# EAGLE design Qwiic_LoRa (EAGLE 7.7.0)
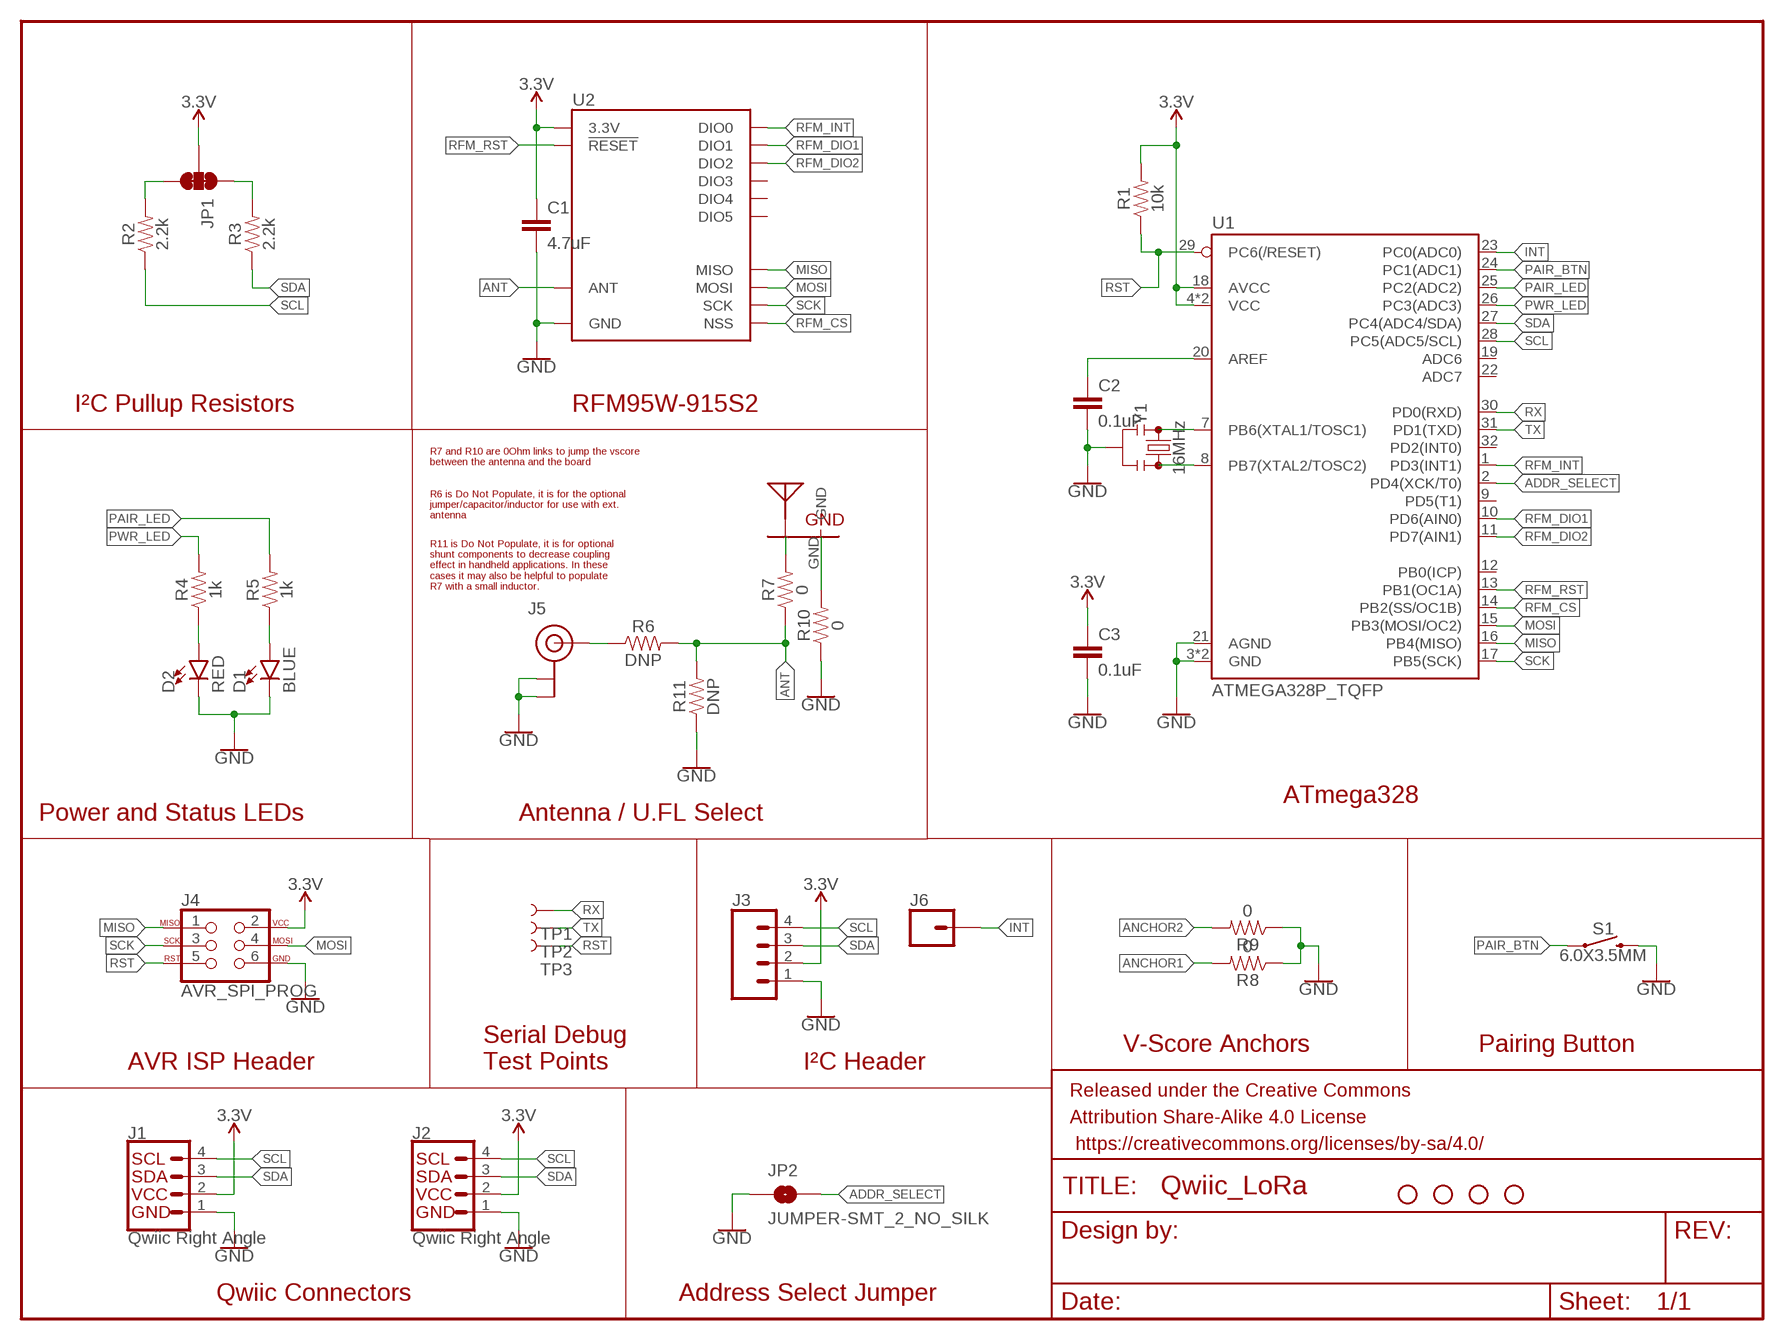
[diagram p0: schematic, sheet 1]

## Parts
C1  4.7uF  4.7UF0603  [0603]
C2  0.1uF  0.1UF-0603-25V-(+80/-20%)  [0603]
C3  0.1uF  0.1UF-0603-25V-(+80/-20%)  [0603]
D1  BLUE  LED-BLUE0603  [LED-0603]
D2  RED  LED-RED0603  [LED-0603]
FRAME1  FRAME-LETTER  [CREATIVE_COMMONS]
H1  STAND-OFF  [STAND-OFF]
H2  STAND-OFF  [STAND-OFF]
H3  STAND-OFF  [STAND-OFF]
H4  STAND-OFF  [STAND-OFF]
J1  Qwiic Right Angle  I2C_STANDARDQWIIC  [1X04_1MM_RA]
J2  Qwiic Right Angle  I2C_STANDARDQWIIC  [1X04_1MM_RA]
J3  CONN_041X04_NO_SILK  [1X04_NO_SILK]
J4  AVR_SPI_PROG  AVR_SPI_PROG_3X2TESTPOINTS  [2X3_TEST_POINTS]
J5  U.FL  [U.FL]
J6  CONN_01PTH_NO_SILK_YES_STOP  [1X01_NO_SILK]
JP1  JUMPER-SMT_3_2-NC_TRACE_SILK  [SMT-JUMPER_3_2-NC_TRACE_SILK]
JP2  JUMPER-SMT_2_NO_SILK  [SMT-JUMPER_2_NO_SILK]
R1  10k  10KOHM-0603-1/10W-1%  [0603]
R2  2.2k  2.2KOHM-0603-1/10W-1%  [0603]
R3  2.2k  2.2KOHM-0603-1/10W-1%  [0603]
R4  1k  1KOHM-0603-1/10W-1%  [0603]
R5  1k  1KOHM-0603-1/10W-1%  [0603]
R6  DNP  RESISTOR0603  [0603]
R7  0  RESISTOR0603  [0603]
R8  0  RESISTOR0603  [0603]
R9  0  RESISTOR0603  [0603]
R10  0  RESISTOR0603  [0603]
R11  DNP  RESISTOR0603  [0603]
S1  6.0X3.5MM  MOMENTARY-SWITCH-SPST-SMD-6.0X3.5MM  [TACTILE_SWITCH_SMD_6.0X3.5MM]
TP1  TEST-POINT3  [PAD.03X.03]
TP2  TEST-POINT3  [PAD.03X.03]
TP3  TEST-POINT3  [PAD.03X.03]
U1  ATMEGA328P_TQFP  [TQFP32-08]
U2  RFM96W  [RFM95/96/97/98W]
U$1  ANTENNA_915MHZ_INVERTED_F  [ANTENNA_INVERTED_F_915MHZ]
Y1  16MHz  RESONATOR-16MHZSMD_3.2X1.3  [RESONATOR-SMD-3.2X1.3]

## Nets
3.3V [3v3]: C1.1 C3.1 J1.2 J2.2 J3.2 J4.2 JP1.2 R1.2 U1.4(VCC) U1.6(VCC) U1.18(AVCC) U2.3.3V
ADDR_SELECT: JP2.2 U1.2(PD4(XCK/T0))
ANCHOR1: R8.2
ANCHOR2: R9.2
ANT: R6.2 R7.1 R11.2 U2.ANT
GND: C1.2 C2.2 C3.2 D1.C D2.C J1.1 J2.1 J3.1 J4.6 J5.1(GND) J5.2(GND) JP2.1 R8.1 R9.1 R10.1 R11.1 S1.2 U1.3(GND) U1.5(GND) U1.21(AGND) U2.GND@1(GND) U2.GND@2(GND) U2.GND@3(GND) Y1.2
INT: J6.1 U1.23(PC0(ADC0))
MISO: J4.1 U1.16(PB4(MISO)) U2.MISO
MOSI: J4.4 U1.15(PB3(MOSI/OC2)) U2.MOSI
N$1: D2.A R4.1
N$2: D1.A R5.1
N$3: C2.1 U1.20(AREF)
N$4: U1.7(PB6(XTAL1/TOSC1)) Y1.1
N$5: U1.8(PB7(XTAL2/TOSC2)) Y1.3
N$6: R7.2 U$1.FEED
N$7: JP1.1 R3.2
N$8: JP1.3 R2.2
N$9: J5.FEED(SIGNAL) R6.1
N$11: R10.2 U$1.GND
PAIR_BTN: S1.1 U1.24(PC1(ADC1))
PAIR_LED: R5.2 U1.25(PC2(ADC2))
PWR_LED: R4.2 U1.26(PC3(ADC3))
RFM_CS: U1.14(PB2(SS/OC1B)) U2.NSS
RFM_DIO1: U1.10(PD6(AIN0)) U2.DIO1
RFM_DIO2: U1.11(PD7(AIN1)) U2.DIO2
RFM_INT: U1.1(PD3(INT1)) U2.DIO0
RFM_RST: U1.13(PB1(OC1A)) U2.!RESET
RST: J4.5 R1.1 TP3.P$1 U1.29(PC6(/RESET))
RX: TP1.P$1 U1.30(PD0(RXD))
SCK: J4.3 U1.17(PB5(SCK)) U2.SCK
SCL: J1.4 J2.4 J3.4 R2.1 U1.28(PC5(ADC5/SCL))
SDA: J1.3 J2.3 J3.3 R3.1 U1.27(PC4(ADC4/SDA))
TX: TP2.P$1 U1.31(PD1(TXD))
Unconnected: U1.9(PD5(T1)) U1.12(PB0(ICP)) U1.19(ADC6) U1.22(ADC7) U1.32(PD2(INT0)) U2.DIO3 U2.DIO4 U2.DIO5

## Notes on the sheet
- I²C Pullup Resistors | RFM95W-915S2
- R7 and R10 are 0Ohm links to jump the vscore 
  between the antenna and the board
- R6 is Do Not Populate, it is for the optional 
  jumper/capacitor/inductor for use with ext.
  antenna
- R11 is Do Not Populate, it is for optional 
  shunt components to decrease coupling 
  effect in handheld applications. In these 
  cases it may also be helpful to populate 
  R7 with a small inductor.
- ATmega328
- Power and Status LEDs | Antenna / U.FL Select
- V-Score Anchors | Pairing Button
- AVR ISP Header
- Serial Debug
  Test Points
- I²C Header
- Qwiic Connectors | Address Select Jumper

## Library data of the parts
C1 = SparkFun-Capacitors:4.7UF: 4.7µF ceramic capacitors; PROD_ID: CAP-08280
C2 C3 = SparkFun-Capacitors:0.1UF: 0.1µF ceramic capacitors; PROD_ID: CAP-00810
D1 = SparkFun-LED:LED-BLUE: Blue SMD LED; PROD_ID: DIO-08575
D2 = SparkFun-LED:LED-RED: Red SMD LED; PROD_ID: DIO-00819
FRAME1 = SparkFun-Aesthetics:FRAME-LETTER: Schematic Frame - Letter
H1-H4 = SparkFun-Hardware:STAND-OFF: Stand Off
J1 J2 = SparkFun-Connectors:I2C_STANDARD: SparkFun I2C Standard Pinout Header SparkFun has standardized on a pinout for all I2C based sensor breakouts. This pinout allows I2C boards to be plugged directly into the headers on Arduino Uno compatible boards, and to be daisy chained easily. Example SparkFun Products: SparkFun Atmospheric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; PROD_ID: CONN-13694
J3 = SparkFun-Connectors:CONN_04: Multi connection point. Often used as Generic Header-pin footprint for 0.1 inch spaced/style header connections On any of the 0.1 inch spaced packages, you can populate with these: Break Away Headers - Straight (PRT-00116) Break Away Male Headers - Right Angle (PRT-00553) Female Headers (PRT-00115)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; PROD_ID: CONN-09696
J4 = SparkFun-Connectors:AVR_SPI_PROG_3X2: AVR ISP 6 Pin This is the reduced ISP connector for AVR programming. Common on Arduino. This footprint will take up less PCB space and can be used with a 10-pin to 6-pin adapter such as SKU: BOB-08508 **Special note about "TEST_POINT" package. The stop mask is on the top side, so if you want your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
J5 = SparkFun-Connectors:U.FL: SMD Antenna Connector - U.FL 2mm height, 3.0mm x 3.0mm receptacle size. SparkFun Products: SparkFun WiFi Shield - ESP8266 SparkFun ESP8266 Thing SparkFun MiniGen - Pro Mini Signal Generator Shield; PROD_ID: CONN-09193; SF_ID: WRL-09144
J6 = SparkFun-Connectors:CONN_01: Single connection point. Often used as Generic Header-pin footprint for 0.1 inch spaced/style header connections
JP1 = SparkFun-Jumpers:JUMPER-SMT_3_2-NC_TRACE: Normally closed trace jumper (2 of 2 connections) This jumper has a trace between all three pads so they are normally closed (NC). Use a razor knife to open the connection(s). For best results follow the IPC guidelines for cutting traces: Cutout at least 0.063 mm (0.005 in). Remove all loose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
JP2 = SparkFun-Jumpers:JUMPER-SMT_2_NO: Normally open jumper
R1 = SparkFun-Resistors:10KOHM: 10kΩ resistor; PROD_ID: RES-00824
R2 R3 = SparkFun-Resistors:2.2KOHM: 2.2kΩ resistor; PROD_ID: RES-08272
R4 R5 = SparkFun-Resistors:1KOHM: 1kΩ resistor; PROD_ID: RES-07856
R6-R11 = SparkFun-Resistors:RESISTOR: Generic Resistor Package
S1 = SparkFun-Switches:MOMENTARY-SWITCH-SPST: Momentary Switch (Pushbutton) - SPST; PROD_ID: SWCH-00815; SF_SKU: COM-08229
TP1-TP3 = SparkFun-Connectors:TEST-POINT: SparkFun Test Points
U1 = SparkFun-IC-Microcontroller:ATMEGA328P_TQFP: Popular 328P in QFP Storefront component: ATmega328 - TQFP (COM-13448) Datasheet SparkFun Products SparkFun RedBoard - Programmed with Arduino (DEV-12757) Arduino Pro Mini 328 - 5V/16MHz (DEV-11113) Arduino Pro Mini 328 - 3.3V/8MHz (DEV-11114) SparkFun OpenLog (DEV-13712) SparkFun MicroView - OLED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; PROD_ID: IC-09069
U2 = SparkX:RFM96W
U$1 = SparkX:ANTENNA_915MHZ_INVERTED_F
Y1 = SparkFun-Clocks:RESONATOR-16MHZ: 16MHz Resonator Digikey Example Frequency: 16MHz Frequency Stability: &plusmn;0.3% Frequency Tolerance: &plusmn;0.5% Capacitance: 15pF SparkFun Products SparkFun OpenLog SparkFun MicroView - OLED Arduino Module; PROD_ID: XTAL-08900

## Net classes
0 default: width 0.152 mm, drill 0.305 mm
1 3v3: width 0.203 mm, drill 0.305 mm

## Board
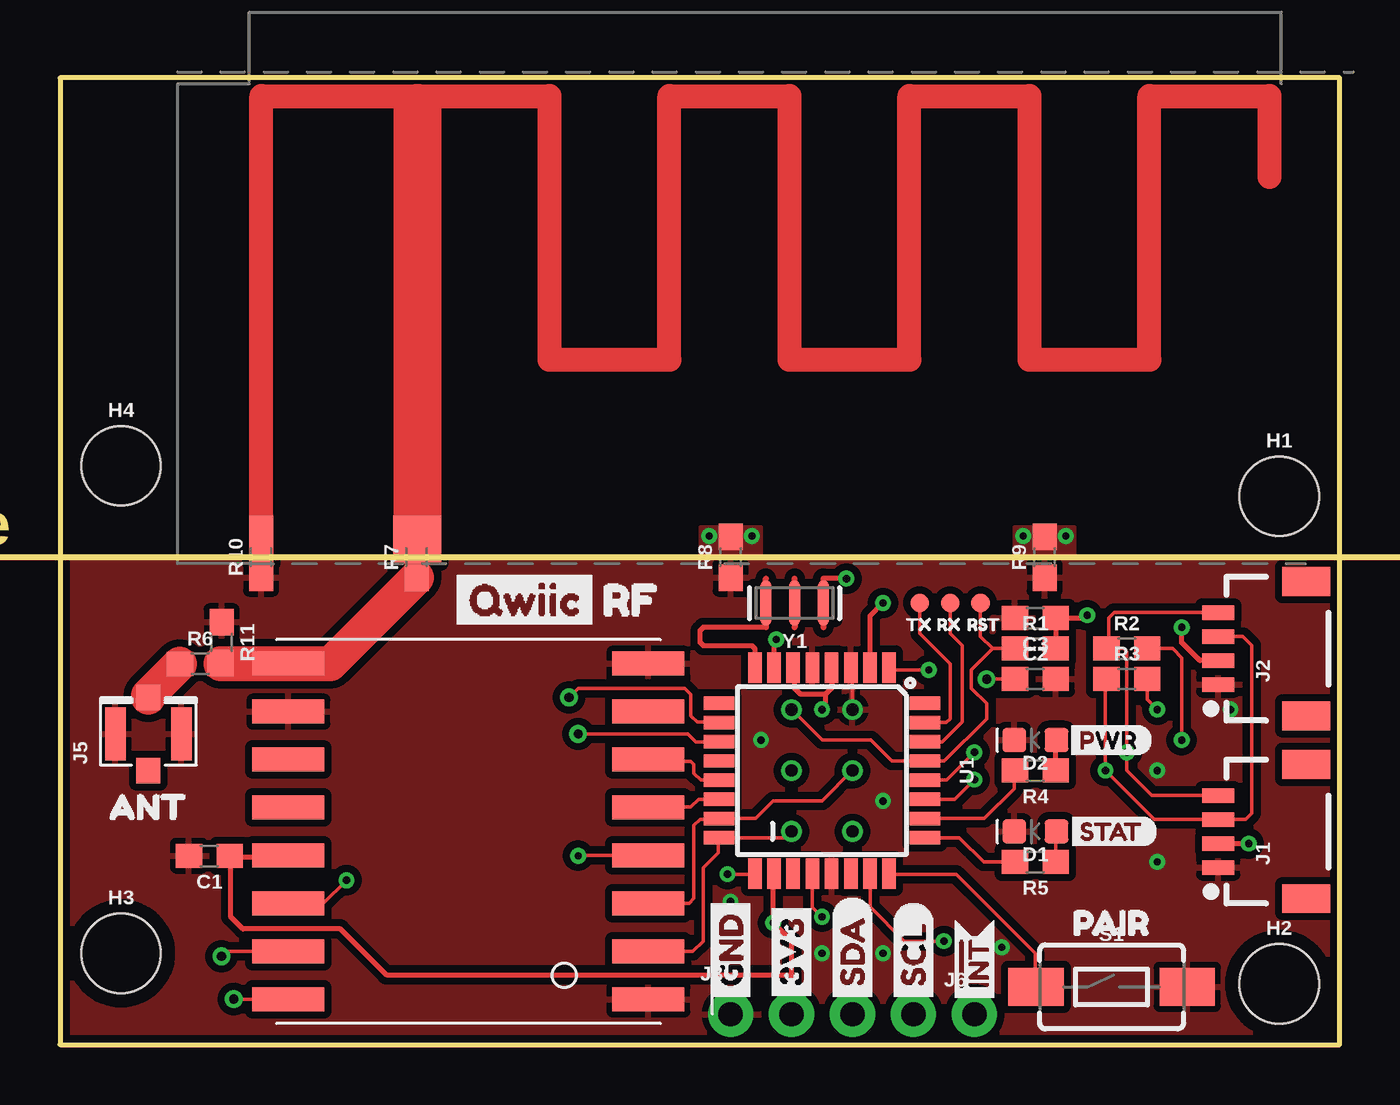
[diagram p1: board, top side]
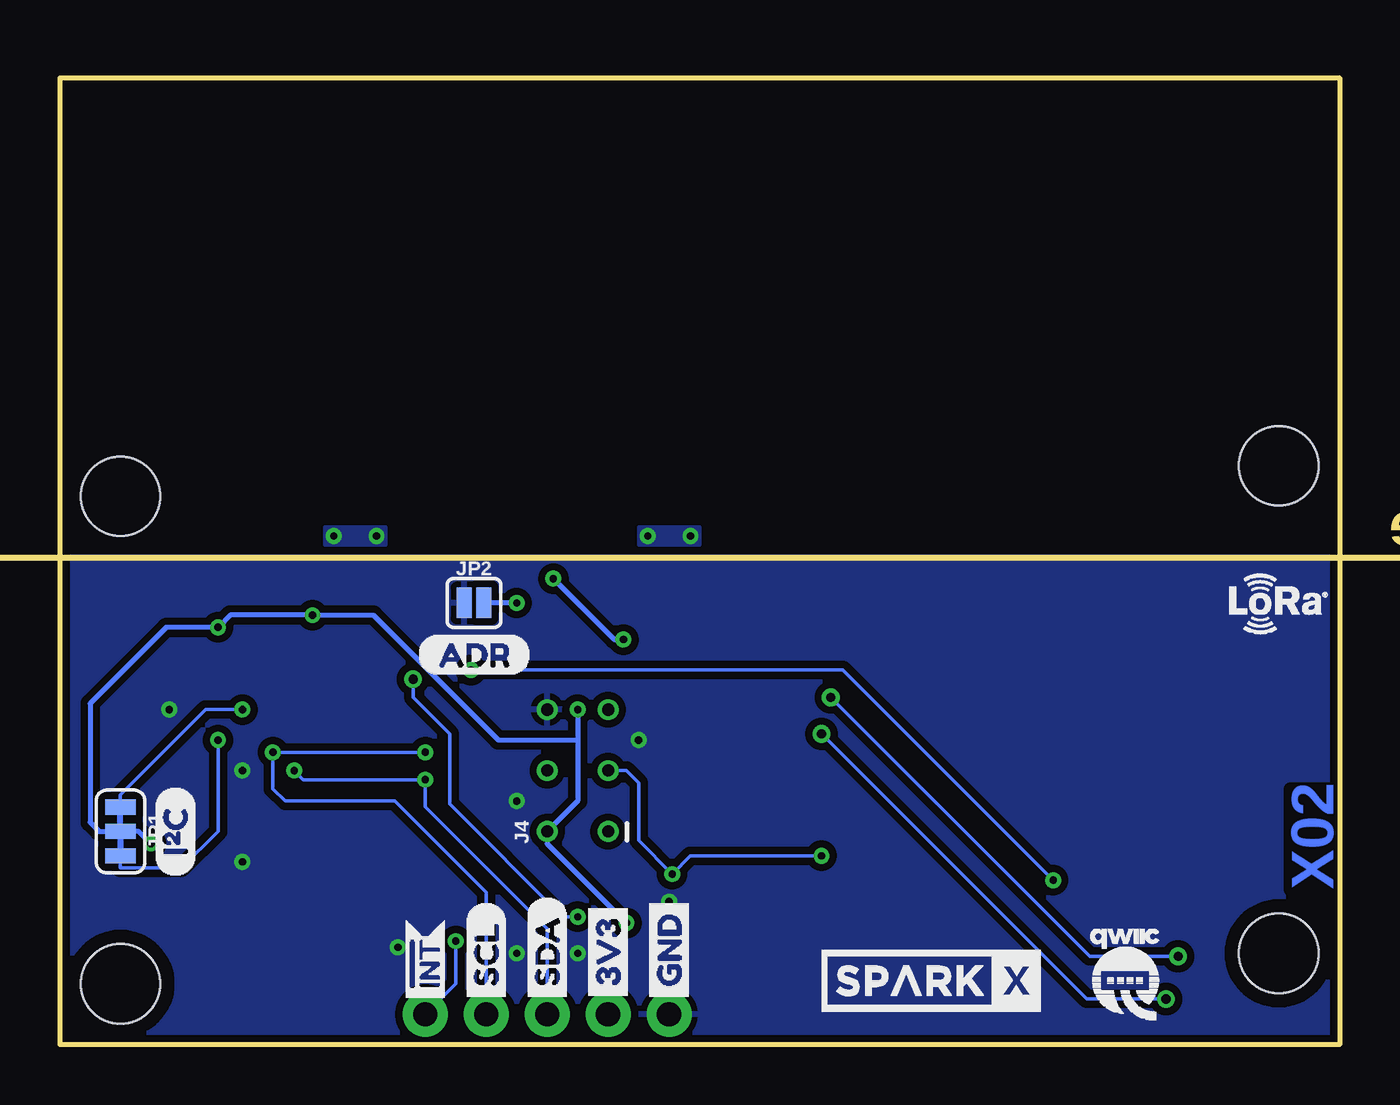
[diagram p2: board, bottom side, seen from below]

Size 53.32 x 40.31 mm. Coordinates in mm from the lower left corner, seen from the top.
Outline: 0,0 53.32,0 53.32,40.31 0,40.31 0,0
Copper layers (1*16): Top 0.035mm / dielectric 1.5mm / Bottom 0.035mm
Design rules "SparkFun-2-layer-PCBWay-LIMIT": minimum track width 6mil, minimum drill 0.3mm, track to track 6mil, track to pad 6mil, pad to pad 6mil, via to via 6mil, smd to smd 6mil, copper to edge 6mil, drill to drill 6mil, minimum pad ring 7mil, minimum via ring 7mil, stop-mask expansion 4mil, vias tented up to drill 25mil, thermal gap 10mil
Milling: 1 lines

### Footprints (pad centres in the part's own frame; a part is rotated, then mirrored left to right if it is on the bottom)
0603 = smd 1.1 x 1: 1 -0.85,0; 2 0.85,0
LED-0603 = smd 1 x 1: A -0.877,0; C 0.877,0
STAND-OFF = hole 3.302: 0,0
1X04_1MM_RA = smd 0.6 x 1.35: 1 -1.5,0; 2 -0.5,0; 3 0.5,0; 4 1.5,0 | smd 1.2 x 2: NC1 2.8,-3.675; NC2 -2.8,-3.675
1X04_NO_SILK = drill 1.016 pad 1.88: 1 0,0; 2 2.54,0; 3 5.08,0; 4 7.62,0
2X3_TEST_POINTS = drill 0.508: 1 -2.54,-1.27; 2 -2.54,1.27; 3 0,-1.27; 4 0,1.27; 5 2.54,-1.27; 6 2.54,1.27
U.FL = smd 2.2 x 0.85: 1 0,1.375; 2 0,-1.375 | smd 1.05 x 1: FEED 1.525,0; NC -1.525,0
1X01_NO_SILK = drill 1.016 pad 1.88: 1 0,0
SMT-JUMPER_3_2-NC_TRACE_SILK = smd 0.635 x 1.27: 1 -1.016,0; 2 0,0; 3 1.016,0
SMT-JUMPER_2_NO_SILK = smd 0.635 x 1.27: 1 -0.406,0; 2 0.406,0
TACTILE_SWITCH_SMD_6.0X3.5MM = smd 2.3 x 1.6: 1 -3.15,0; 2 3.15,0
PAD.03X.03 = smd 0.762 x 0.762: P$1 0,0
TQFP32-08 = smd 1.27 x 0.559: 1 -4.293,2.8; 2 -4.293,2; 3 -4.293,1.2; 4 -4.293,0.4; 5 -4.293,-0.4; 6 -4.293,-1.2; 7 -4.293,-2; 8 -4.293,-2.8; 17 4.293,-2.8; 18 4.293,-2; 19 4.293,-1.2; 20 4.293,-0.4; 21 4.293,0.4; 22 4.293,1.2; 23 4.293,2; 24 4.293,2.8 | smd 0.559 x 1.27: 9 -2.8,-4.293; 10 -2,-4.293; 11 -1.2,-4.293; 12 -0.4,-4.293; 13 0.4,-4.293; 14 1.2,-4.293; 15 2,-4.293; 16 2.8,-4.293; 25 2.8,4.293; 26 2,4.293; 27 1.2,4.293; 28 0.4,4.293; 29 -0.4,4.293; 30 -1.2,4.293; 31 -2,4.293; 32 -2.8,4.293
RFM95/96/97/98W = smd 3 x 1: 3.3V 7.5,1; !RESET -7.5,-3; ANT 7.5,-7; DIO0 7.5,3; DIO1 7.5,5; DIO2 7.5,7; DIO3 7.5,-3; DIO4 7.5,-1; DIO5 -7.5,-5; GND@1 -7.5,7; GND@2 -7.5,-7; GND@3 7.5,-5; MISO -7.5,5; MOSI -7.5,3; NSS -7.5,-1; SCK -7.5,1
ANTENNA_INVERTED_F_915MHZ = smd 2 x 2: FEED 6,2 | smd 1 x 2: GND -0.5,2
RESONATOR-SMD-3.2X1.3 = smd 0.45 x 1.905: 1 -1.2,0; 2 0,0; 3 1.2,0

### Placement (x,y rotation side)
C1  6.22,7.87 180 top
C2  40.64,15.24 0 top
C3  40.64,17.78 180 top
D1  40.64,8.89 180 top
D2  40.64,12.7 180 top
FRAME1  not placed on the board
H1  50.8,22.86 0 top
H2  50.8,2.54 0 top
H3  2.54,3.81 0 top
H4  2.54,24.13 0 top
J1  48.26,8.89 90 top
J2  48.26,16.51 90 top
J3  27.94,1.27 0 top
J4  31.75,11.43 90 bottom
J5  3.68,12.95 90 top
J6  38.1,1.27 0 top
JP1  50.8,8.89 270 bottom
JP2  36.07,18.41 0 bottom
R1  40.64,16.51 0 top
R2  44.45,16.51 0 top
R3  44.45,15.24 0 top
R4  40.64,11.43 180 top
R5  40.64,7.62 180 top
R6  5.84,15.88 0 top
R7  14.86,20.32 90 top
R8  27.94,20.32 90 top
R9  41.02,20.32 90 top
R10  8.38,20.32 90 top
R11  6.73,16.76 270 top
S1  43.81,2.41 0 top
TP1  37.08,18.41 0 top
TP2  35.81,18.41 0 top
TP3  38.35,18.41 0 top
U1  31.75,11.43 270 top
U2  17.02,8.89 180 top
U$1  8.89,19.05 0 top
U$2  [ANT0]  1.14,9.91 0 top
U$3  [PAIR1]  41.27,5.08 0 top
U$4  [SDA-[)]  33.02,1.52 90 top
U$5  [SCL-[)]  35.56,1.52 90 top
U$6  [GND-04]  27.94,1.52 90 top
U$7  [3V3-04]  30.48,1.52 90 top
U$8  [PWR1]  41.78,12.7 0 top
U$9  [STAT2]  41.78,8.89 0 top
U$10  [QWIIC-LOGO-SMALL]  9.02,2.92 0 bottom
U$11  [TX1]  34.8,17.53 0 top
U$12  [INT#-[<]  38.1,1.27 90 top
U$13  [SPARKX-MEDIUM]  17.02,2.67 0 bottom
U$14  [ADR-()]  38.48,16.26 0 bottom
U$15  [RF1]  21.46,18.54 0 top
U$16  [QWIIC0]  15.88,18.54 0 top
U$17  [LORA_MARK#PNG]  2.67,18.41 0 bottom
U$18  [GND-04]  27.94,1.52 90 top
U$19  [GND-04]  27.94,1.52 90 bottom
U$20  [3V3-04]  30.48,1.52 90 top
U$21  [3V3-04]  30.48,1.52 90 bottom
U$22  [SDA-[)]  33.02,1.52 90 bottom
U$23  [SCL-[)]  35.56,1.52 90 bottom
U$24  [INT#-[<]  38.1,1.27 90 bottom
U$25  [I_SUPER2_C-()-04]  48.51,6.99 90 bottom
U$26  [PRODUCTION_INSTRUCTIONS]  not placed on the board
U$27  [RX0]  36.07,17.53 0 top
U$28  [RST2]  37.34,17.53 0 top
Y1  30.61,18.41 180 top

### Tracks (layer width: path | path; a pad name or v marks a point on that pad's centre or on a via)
3.3V  (via drill 0.3)
  Top 0.203: J3.2 30.48,2.92 | 30.48,2.92 30.48,4.32 v29.72,5.08 29.72,7.11 U1.18 | 30.48,2.92 13.59,2.92 11.68,4.83 7.62,4.83 7.11,5.33 7.11,7.83 | J1.2 v49.52,8.39 v49.53,8.38 | J2.2 47.49,16.01 46.74,16.76 v46.74,17.4 | U1.4 32.15,14.88 31.88,14.61 | 31.88,14.61 30.86,14.61 30.61,14.86 30.61,15.67 U1.6 | 31.88,14.61 31.88,14.1 v31.75,13.97 | 41.53,16.55 R1.2 C3.1 42.67,17.78 v42.8,17.91 | 7.11,7.83 C1.1 | 7.11,7.83 9.46,7.83 U2.3.3V
  Bottom 0.203: v49.53,8.38 50.04,8.89 JP1.2 51.69,8.89 52.07,9.27 52.07,14.22 48.9,17.4 v46.74,17.4 46.23,17.91 v42.8,17.91 40.26,17.91 35.05,12.7 31.75,12.7 | v29.72,5.08 33.02,8.38 J4.2 31.75,10.16 31.75,12.7 | v31.75,13.97 31.75,12.7
ADDR_SELECT  (via drill 0.3)
  Top 0.203: U1.2 33.75,17.88 v34.29,18.41
  Bottom 0.203: v34.29,18.41 JP2.2
ANCHOR1  (via drill 0.3)
  other vias: 27.05,21.21 28.83,21.21
  pour Top (isolate 0.305, no thermals): 26.67,21.59 29.21,21.59 29.21,20.32 26.67,20.32
  pour Bottom (isolate 0.305, no thermals): 26.67,21.59 29.21,21.59 29.21,20.83 26.67,20.83
ANCHOR2  (via drill 0.3)
  other vias: 40.13,21.21 41.91,21.21
  pour Bottom (isolate 0.305, no thermals): 39.75,21.59 42.29,21.59 42.29,20.83 39.75,20.83
  pour Top (isolate 0.305, no thermals): 39.75,21.59 42.29,21.59 42.29,20.32 39.75,20.32
ANT
  Top 0.254: R11.2 R6.2
  Top 1.448: 6.71,15.89 U2.ANT 11.28,15.89 | R6.2 11.26,15.88 11.28,15.89 | 11.28,15.89 R7.1
GND  (via drill 0.3)
  Top 0.152: J4.6 33.02,15.65 U1.3
  other vias: 48.77,13.97 29.21,12.7 27.94,5.97 45.72,11.43 34.29,10.16 45.72,7.62 31.75,3.81 34.29,3.81 39.24,4.06
  pour Bottom (isolate 0.305): 0,20.32 53.34,20.32 53.34,0 0,0
  pour Top (isolate 0.305): 0,20.32 53.34,20.32 53.34,0 0,0
INT  (via drill 0.3)
  Top 0.152: U1.23 33.75,5.75 35.18,4.32 v36.83,4.32
  Bottom 0.152: v36.83,4.32 36.83,2.54 J6.1
MISO
  Top 0.152: J4.1 30.22,8.63 U1.16 27.43,8.61 27.43,8 26.8,7.37 26.8,4.32 26.37,3.89 U2.MISO
MOSI
  Top 0.152: J4.4 31.75,10.16 29.72,10.16 28.99,9.43 U1.15 27.43,9.4 26.67,9.4 26.42,9.14 26.42,6.1 26.21,5.89 U2.MOSI
N$1
  Top 0.152: R4.1 41.49,11.4
  Top 0.203: 41.49,11.4 41.49,12.67 D2.A
N$2
  Top 0.152: R5.1 41.49,8.86 D1.A
N$3  (via drill 0.3, 0.38)
  Top 0.152: U1.20 31.35,5.73 v31.75,5.33 | 39.75,15.2 C2.1 v38.61,15.24
  Bottom 0.152: v31.75,5.33 32.38,5.33 37.08,10.03 37.08,12.95 38.61,14.48 v38.61,15.24
N$4  (via drill 0.3)
  Top 0.203: U1.7 29.75,16.8 v29.84,16.89 | v32.77,19.43 31.81,19.43
  Bottom 0.203: v29.84,16.89 30.23,16.89 v32.77,19.43
N$5
  Top 0.152: U1.8
  Top 0.203: U1.8 28.96,16.51 28.83,16.64 26.8,16.64 26.67,16.76 26.67,17.27 26.8,17.4 29.41,17.4
N$6
  Top 0.203: R7.2 14.86,21.08 U$1.FEED
N$7  (via drill 0.3)
  Top 0.152: R3.2 45.3,14.39 v45.72,13.97
  Bottom 0.152: v45.72,13.97 47.24,13.97 50.8,10.41 JP1.1
N$8  (via drill 0.3)
  Top 0.152: R2.2 46.35,16.51 46.74,16.13 v46.74,12.7
  Bottom 0.152: v46.74,12.7 46.74,8.89 48.26,7.37 50.8,7.37 JP1.3
N$9
  Top 1.448: J5.FEED 3.68,14.57 R6.1
N$11
  Top 0.254: U$1.GND R10.2
PAIR_BTN
  Top 0.152: U1.24 34.58,7.11 37.34,7.11 40.64,3.81 40.64,2.44 S1.1
PAIR_LED
  Top 0.152: U1.25 37.47,8.63 38.48,7.62 R5.2
PWR_LED
  Top 0.152: U1.26 38.51,9.43 39.75,10.67 39.75,11.39 R4.2
RFM_CS
  Top 0.152: U1.14 26.61,10.23 26.29,9.91 24.53,9.91 U2.NSS
RFM_DIO1  (via drill 0.38)
  Top 0.152: U2.DIO1 6.94,3.89 v6.73,3.68 | v21.21,14.48 21.59,14.86 26.04,14.86 26.29,14.61 26.29,13.72 26.54,13.46 27.43,13.46 U1.10
  Bottom 0.152: v6.73,3.68 10.41,3.68 v21.21,14.48
RFM_DIO2  (via drill 0.38)
  Top 0.152: U2.DIO2 7.25,1.89 v7.24,1.91 | v21.59,12.95 26.16,12.95 26.49,12.63 U1.11
  Bottom 0.152: v7.24,1.91 10.54,1.91 v21.59,12.95
RFM_INT  (via drill 0.3)
  Top 0.152: v11.94,6.86 10.97,5.89 U2.DIO0 | v36.2,15.62 34.65,15.62 U1.1
  Bottom 0.152: v11.94,6.86 20.7,15.62 v36.2,15.62
RFM_RST
  Top 0.152: U1.13 26.69,11.03 26.42,11.3 26.42,11.68 26.29,11.81 24.6,11.81 U2.!RESET
RST
  Top 0.152: J4.5 31.75,12.7 33.78,12.7 34.65,11.83 U1.29 36.85,11.83 38.61,13.59 38.61,14.22 37.97,14.86 37.97,15.62 38.86,16.51 | 38.86,16.51 R1.1 | TP3.P$1 38.35,17.02 38.86,16.51
RX
  Top 0.152: U1.30 36.76,12.63 37.59,13.46 37.59,16.64 37.08,17.14 TP1.P$1
SCK  (via drill 0.3)
  Top 0.152: v21.59,7.87 21.61,7.89 U2.SCK | v27.81,7.11 28.93,7.11 U1.17
  Bottom 0.152: v21.59,7.87 27.05,7.87 v27.81,7.11 29.21,8.51 29.21,10.92 29.72,11.43 J4.3
SCL  (via drill 0.3)
  Top 0.152: J1.4 45.49,10.39 44.45,11.43 v44.45,12.19 44.45,16.38 44.32,16.51 R2.1 43.69,16.6 43.69,17.78 43.92,18.01 J2.4 | U1.28 36.94,11.03 v38.1,12.19
  Bottom 0.152: v38.1,12.19 v44.45,12.19 44.45,10.67 43.94,10.16 39.37,10.16 35.56,6.35 J3.4
SDA  (via drill 0.3)
  Top 0.152: 43.56,15.2 v43.56,11.43 45.6,9.39 J1.3 49.4,9.4 49.66,9.65 49.66,16.64 49.28,17.01 J2.3 | U1.27 37.28,10.23 v38.1,11.05
  Top 0.203: 43.56,15.2 R3.1
  Bottom 0.152: v43.56,11.43 43.18,11.05 v38.1,11.05 38.1,9.91 33.02,4.83 J3.3
TX
  Top 0.152: U1.31 36.92,13.43 37.08,13.59 37.08,15.88 35.81,17.14 TP2.P$1

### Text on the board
Bottom: X02
Milling: vscore
tDocu: 0.8mm Thickness PCB | RFM95W / 915MHz | NPoole 2018

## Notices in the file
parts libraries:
SparkFun-Switches: Licensing: Creative Commons ShareAlike 4.0 International - https://creativecommons.org/licenses/by-sa/4.0
SparkFun-Aesthetics: Released under the Creative Commons Attribution Share-Alike 4.0 License
SparkFun-Aesthetics: https://creativecommons.org/licenses/by-sa/4.0
